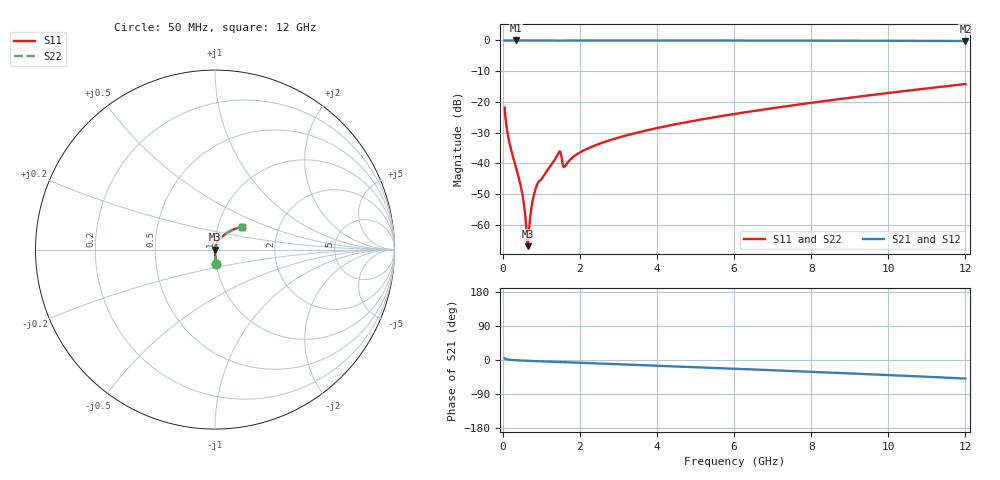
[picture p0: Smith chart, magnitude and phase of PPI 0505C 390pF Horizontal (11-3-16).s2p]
# MHz S MA R 50
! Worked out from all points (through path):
!   1601 points, 50 MHz to 12 GHz, reference 50 ohm
!   highest |S21| = 0.00 dB at 333.8 MHz (marker M1); lowest = -0.2 dB at 12 GHz (marker M2)
!   group delay of S21, straight-line fit = 11.3 ps
!   lowest |S11| = -67.0 dB at 647.5 MHz (marker M3), VSWR 1.00, Z = 50 - j0.00623 ohm
!   |S11| at or under -10 dB: start of sweep to end of sweep
!   |S22| runs from -67.0 to -14.2 dB; largest |S21 - S12| = 0
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50  0.08077 -85.4  0.9965 4.5  0.9965 4.5  0.08077 -85.4
176.9688  0.02136 -88.6  0.9995 0.6  0.9995 0.6  0.02136 -88.6
333.8125  0.009056 -88.4  0.9996 -0.6  0.9996 -0.6  0.009056 -88.4
498.125  0.003456 -84.9  0.9996 -1.4  0.9996 -1.4  0.003456 -84.9
550.4062  0.002179 -80.9  0.9996 -1.7  0.9996 -1.7  0.002179 -80.9
610.1562  0.0009203 -64.2  0.9995 -1.9  0.9995 -1.9  0.0009203 -64.2
647.5  0.0004468 -8.0  0.9995 -2.1  0.9995 -2.1  0.0004468 -8.0
684.8438  0.0008297 53.8  0.9995 -2.3  0.9995 -2.3  0.0008297 53.8
752.0625  0.002017 72.6  0.9994 -2.6  0.9994 -2.6  0.002017 72.6
804.3438  0.002962 75.7  0.9994 -2.8  0.9994 -2.8  0.002962 75.7
931.3125  0.005003 72.3  0.9987 -3.3  0.9987 -3.3  0.005003 72.3
1446.656  0.01468 69.3  0.996 -5.5  0.996 -5.5  0.01468 69.3
1491.469  0.0155 54.7  0.9921 -5.6  0.9921 -5.6  0.0155 54.7
1573.625  0.008884 52.2  0.9951 -5.6  0.9951 -5.6  0.008884 52.2
1618.438  0.008969 66.1  0.9971 -5.8  0.9971 -5.8  0.008969 66.1
2044.156  0.0155 79.2  0.9989 -7.5  0.9989 -7.5  0.0155 79.2
2835.844  0.02435 77.4  0.9987 -10.6  0.9987 -10.6  0.02435 77.4
4038.312  0.03784 73.3  0.9981 -15.3  0.9981 -15.3  0.03784 73.3
6025  0.0637 65.9  0.9965 -23.1  0.9965 -23.1  0.0637 65.9
8019.156  0.0968 58.0  0.9935 -31.2  0.9935 -31.2  0.0968 58.0
10013.31  0.1398 49.6  0.988 -39.8  0.988 -39.8  0.1398 49.6
12000  0.1949 40.5  0.9783 -48.9  0.9783 -48.9  0.1949 40.5
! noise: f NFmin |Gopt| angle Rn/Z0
50  0.0003106  0.833  0.241  0.0003926
1372  0.004664  0.7148  4.436  0.003224
2701  0.004959  0.53  8.52  0.001849
4031  0.006473  0.4819  12.48  0.00211
5360  0.007967  0.4541  16.3  0.002401
6682  0.009433  0.4365  19.96  0.002698
8012  0.01092  0.4259  23.48  0.003013
9341  0.01244  0.421  26.86  0.003356
1.067e+04  0.01403  0.4209  30.09  0.003739
1.2e+04  0.01571  0.425  33.19  0.004175
